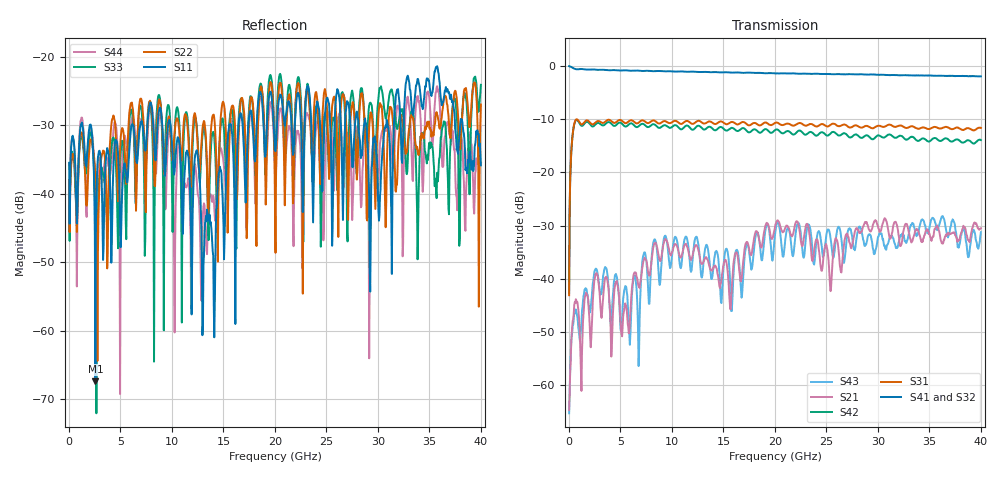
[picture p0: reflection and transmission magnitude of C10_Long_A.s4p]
!Keysight Technologies,N5245A,MY52451697,A.10.60.06
!Date: Wednesday, October 06, 2021 18:59:08
!Correction: S11(Full 4 Port(1,2,3,4))
!S12(Full 4 Port(1,2,3,4))
!S13(Full 4 Port(1,2,3,4))
!S14(Full 4 Port(1,2,3,4))
!S21(Full 4 Port(1,2,3,4))
!S22(Full 4 Port(1,2,3,4))
!S23(Full 4 Port(1,2,3,4))
!S24(Full 4 Port(1,2,3,4))
!S31(Full 4 Port(1,2,3,4))
!S32(Full 4 Port(1,2,3,4))
!S33(Full 4 Port(1,2,3,4))
!S34(Full 4 Port(1,2,3,4))
!S41(Full 4 Port(1,2,3,4))
!S42(Full 4 Port(1,2,3,4))
!S43(Full 4 Port(1,2,3,4))
!S44(Full 4 Port(1,2,3,4))
!S4P File: Measurements: <S11,S12,S13,S14>,
!<S21,S22,S23,S24>,
!<S31,S32,S33,S34>,
!<S41,S42,S43,S44>:
# Hz S  dB  R 50
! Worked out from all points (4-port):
!   801 points, 10 MHz to 40 GHz, reference 50 ohm
!   strongest paths, dB at 10 MHz, 10.01 GHz, 20 GHz, 30 GHz, 40 GHz:
!     S41: 0.0, -1.0, -1.4, -1.6, -1.9
!     S32: 0.0, -1.0, -1.4, -1.7, -2.0
!     S31: -43.1, -10.6, -10.7, -11.2, -11.6
!     S42: -42.6, -11.4, -12.0, -13.0, -13.9
!     S21: -64.7, -35.1, -30.2, -30.1, -30.5
!     S43: -65.3, -35.6, -31.7, -32.2, -31.2
!   lowest |S11| = -67.4 dB at 2.559 GHz (marker M1), VSWR 1.00, Z = 50 + j0.0347 ohm
!   |S11| at or under -10 dB: start of sweep to end of sweep
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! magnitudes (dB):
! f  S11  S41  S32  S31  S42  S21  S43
! 10 MHz  -35.5  0.0  0.0  -43.1  -42.6  -64.7  -65.3
! 509.9 MHz  -33.1  -0.5  -0.5  -10.9  -10.9  -44.9  -46.2
! 2.559 GHz  -67.4  -0.7  -0.7  -10.6  -11.0  -39.3  -38.2
! 8.708 GHz  -28.1  -0.9  -0.9  -10.8  -11.6  -35.7  -39.0
! 14.06 GHz  -56.1  -1.1  -1.1  -10.8  -12.0  -37.9  -37.2
! 18.56 GHz  -25.1  -1.3  -1.3  -11.1  -12.5  -33.5  -33.9
! 40 GHz  -35.8  -1.9  -2.0  -11.6  -13.9  -30.5  -31.2
